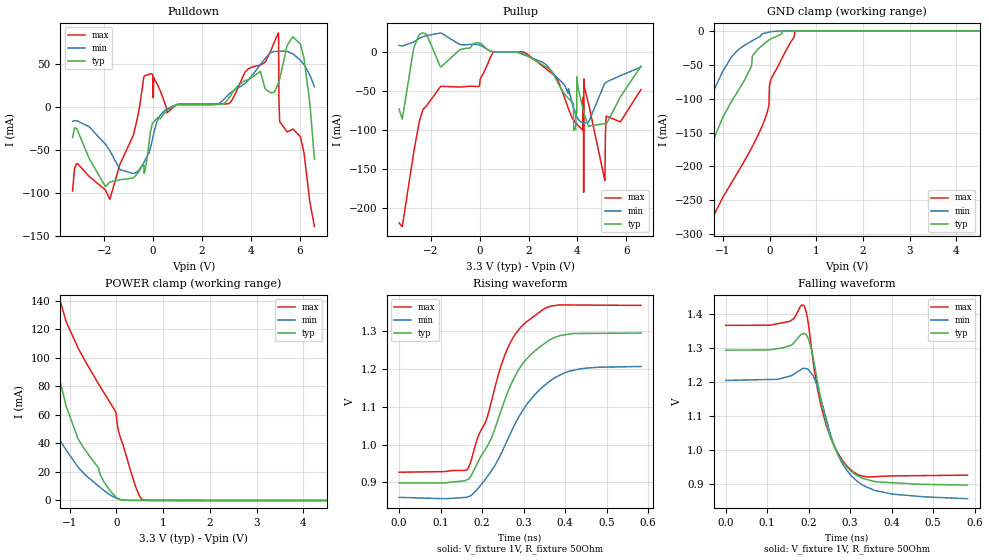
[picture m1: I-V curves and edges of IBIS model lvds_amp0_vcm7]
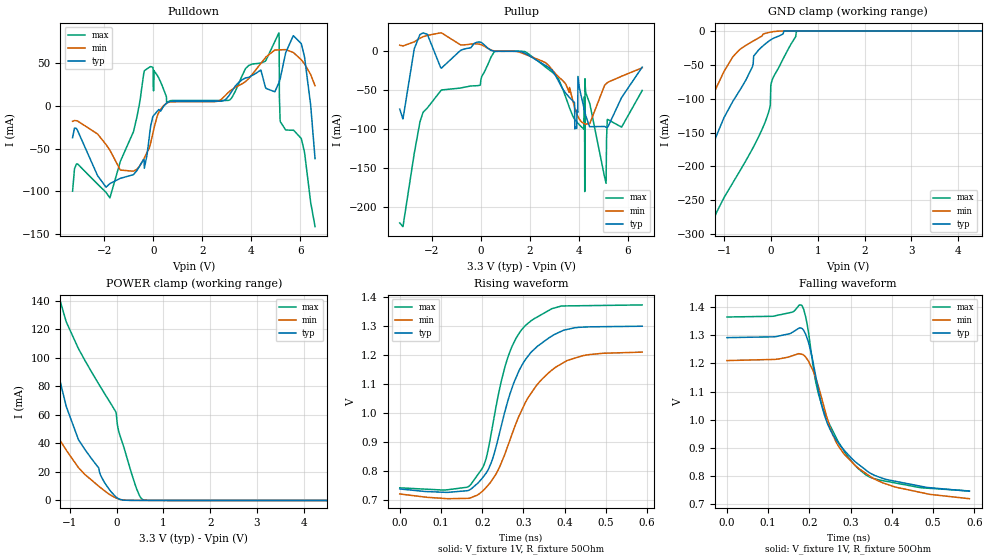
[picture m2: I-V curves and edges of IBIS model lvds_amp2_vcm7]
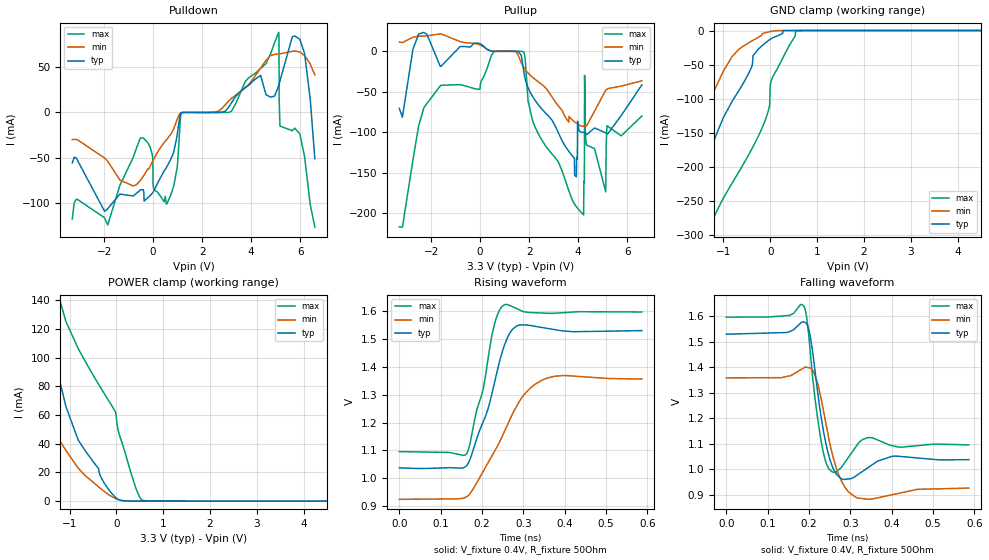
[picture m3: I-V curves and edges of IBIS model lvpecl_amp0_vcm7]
|Texas Instruments Incorporated
| LMK5C33XXX Network Clock Generator/Synchronizer
| Marketing part#   Digital Voltage Range   Package-type   #pins
| LMK5C33216   3.135-3.465V   QFN   64
[IBIS Ver] 4.1
[File name] lmk5c33216.ibs
[File Rev] 1.2
[Date] 2020-10-04
[Source]
| Texas Instruments Incorporated.
| 12500 TI Blvd
| Dallas, TX -75243
[Notes] Revision History:
| Rev 1.2: 2020-10-04, MSG
| - Added models GPIO, XO, INX, I2C for Input/Output pins
| Rev 1.1: 2020-09-02, TT
| - Updated pin names to match datasheet.
| - Corrected typo for LVPECL amplitude names.
| - Note: When AC coupling LVPECL, use small capacitors for best simulation results.
| - Note: When using HSDS, (HSDS_AMP0_VCM7_B0, HSDS_AMP3_VCM7_B0, HSDS_AMP3_VCM7_B1.
| 	- A large deviation in starting voltage may be observed due.
| 	- Setting the common mode voltage may resolve this simulation issue.
| Rev 1.0: 2020-08-25
| - Initial version of the model
| - Model generated from simulations in TISPICE/SPECTRE
| - C_comp although listed in numerical order of value are
| obtained from varying PVT conditions. For PVT conditions for
| each specific value refer the buffer description under
| respective [Model]. IBIS model user is responsible for using
| appropriate C_comp to simulate for Signal Integrity.
| - Warnings regarding combined Non-monotonicity of various models have been
| reviewed and considered minor and can be ignored.
|**** Explanation of [Model Selector]*****************
| - Model names contain the protocol name and
| - amplitude setting 0 to 3 for higher swing
| - DC Shift setting is set to 7
| - HSDS Mode Boost can be on or off as per user requirements
| - lvds_amp0_vcm7 means LVDS MODE, AMPLITUDE 0, DC SHIFT 7
| - hsds_amp0_vcm7_b0 means HSDS MODE, AMPLITUDE 0, DC SHIFT 7, BOOST OFF
| - hsds_amp0_vcm7_b1 means HSDS MODE, AMPLITUDE 0, DC SHIFT 7, BOOST ON
| - cml_amp0_vcm7 means CML MODE, AMPLITUDE 0, DC SHIFT 7
[Disclaimer]
| This model is designed as an aid for customers of Texas Instruments.
| TI and its licensors and suppliers make no warranties, either expressed
| or implied, with respect to this model, including the warranties of
| merchantability or fitness for a particular purpose. The model is
| provided solely on an "as is" basis. The entire risk as to its quality
| and performance is with the customer.
| This model is subject to change without notice. Texas Instruments
| Incorporated is not responsible for updating this model.
[Copyright]
(C) Copyright 2020 Texas Instruments Incorporated. All rights reserved.
| LMK5C33216 (per package)
[Component] LMK5C33216
[Manufacturer] Texas Instruments Incorporated
[Package] |VQFN 64-pin
|   typ   min   max
R_pkg   0.067   0.027   0.083
L_pkg   0.937nH   0.593nH   1.143nH
C_pkg   0.144pF   0.126pF   0.200pF
[Pin]  signal_name 		model_name   R_pin   L_pin   C_pin
1	VDDO_01		power		NA	NA	NA
2	OUT0_P		multimode_out	NA	NA	NA
3	OUT0_N		multimode_out	NA	NA	NA
4	OUT1_P		multimode_out	NA	NA	NA
5	OUT1_N		multimode_out	NA	NA	NA
6	LF1		nc		NA	NA	NA
7	CAP_APLL1		nc		NA	NA	NA
8	VDD_APLL1_XO		power		NA	NA	NA
9	XO_P		xo		NA	NA	NA
10	GPIO2		GPIO		NA	NA	NA
11	VDDO_23		power		NA	NA	NA
12	OUT2_P		multimode_out	NA	NA	NA
13	OUT2_N		multimode_out	NA	NA	NA
14	OUT3_N		multimode_out	NA	NA	NA
15	OUT3_P		multimode_out	NA	NA	NA
16	SDIO		I2C		NA	NA	NA
17	SCK		I2C		NA	NA	NA
18	SCS_ADD_TOD		I2C		NA	NA	NA
19	LF2		nc		NA	NA	NA
20	CAP3_APLL2	nc		NA	NA	NA
21	CAP2_APLL2	nc		NA	NA	NA
22	CAP1_APLL2		nc		NA	NA	NA
23	VDD_APLL2		power		NA	NA	NA
24	OUT5_P		multimode_out	NA	NA	NA
25	OUT5_N		multimode_out	NA	NA	NA
26	OUT4_N		multimode_out	NA	NA	NA
27	OUT4_P		multimode_out	NA	NA	NA
28	VDDO_4567		power		NA	NA	NA
29	OUT6_P		multimode_out	NA	NA	NA
30	OUT6_N		multimode_out	NA	NA	NA
31	OUT7_N		multimode_out	NA	NA	NA
32	OUT7_P		multimode_out	NA	NA	NA
33	VDD_IN0		power		NA	NA	NA
34	IN0_P		INX		NA	NA	NA
35	IN0_N		INX		NA	NA	NA
36	PDN#		I2C		NA	NA	NA
37	VDD_IN1		power		NA	NA	NA
38	IN1_N		INX		NA	NA	NA
39	IN1_P		INX		NA	NA	NA
40	CAP_DIG		nc		NA	NA	NA
41	VDD_DIG		power		NA	NA	NA
42	OUT14_P		multimode_out	NA	NA	NA
43	OUT14_N		multimode_out	NA	NA	NA
44	VDDO_OUT1415		power		NA	NA	NA
45	OUT15_N		multimode_out	NA	NA	NA
46	OUT15_P		multimode_out	NA	NA	NA
47	VDD_APLL3		power		NA	NA	NA
48	CAP_APLL3		nc		NA	NA	NA
49	LF3		nc		NA	NA	NA
50	GPIO0		GPIO		NA	NA	NA
51	OUT8_P		multimode_out	NA	NA	NA
52	OUT8_N		multimode_out	NA	NA	NA
53	OUT9_N		multimode_out	NA	NA	NA
54	OUT9_P		multimode_out	NA	NA	NA
55	VDDO_8910111213	power		NA	NA	NA
56	OUT10_P		multimode_out	NA	NA	NA
57	OUT10_N		multimode_out	NA	NA	NA
58	OUT11_N		multimode_out	NA	NA	NA
59	OUT11_P		multimode_out	NA	NA	NA
60	OUT12_P		multimode_out	NA	NA	NA
61	OUT12_N		multimode_out	NA	NA	NA
62	OUT13_N		multimode_out	NA	NA	NA
63	OUT13_P		multimode_out	NA	NA	NA
64	GPIO1		GPIO		NA	NA	NA
[Diff pin]  inv_pin  vdiff  tdelay_typ  tdelay_min  tdelay_max
2   3   0.0   0.0s   0.0s   0.0s
4   5   0.0   0.0s   0.0s   0.0s
12   13   0.0   0.0s   0.0s   0.0s
14   15   0.0   0.0s   0.0s   0.0s
24   25   0.0   0.0s   0.0s   0.0s
26   27   0.0   0.0s   0.0s   0.0s
29   30   0.0   0.0s   0.0s   0.0s
31   32   0.0   0.0s   0.0s   0.0s
34   35   0.2   0.0s   0.0s   0.0s
38   39   0.2   0.0s   0.0s   0.0s
42   43   0.0   0.0s   0.0s   0.0s
45   46   0.0   0.0s   0.0s   0.0s
51   52   0.0   0.0s   0.0s   0.0s
53   54   0.0   0.0s   0.0s   0.0s
56   57   0.0   0.0s   0.0s   0.0s
58   59   0.0   0.0s   0.0s   0.0s
60   61   0.0   0.0s   0.0s   0.0s
62   63   0.0   0.0s   0.0s   0.0s
|CML MODE available only on pins Out4 & 6 and not available on any other pins
[Model Selector] multimode_out
lvds_amp0_vcm7 Amplitude setting 0, DC shift setting 7
lvds_amp1_vcm7 Amplitude setting 1, DC shift setting 7
lvds_amp2_vcm7 Amplitude setting 2, DC shift setting 7
lvds_amp3_vcm7 Amplitude setting 3, DC shift setting 7
lvpecl_amp0_vcm7 Amplitude setting 0, DC shift setting 7
lvpecl_amp1_vcm7 Amplitude setting 1, DC shift setting 7
lvpecl_amp2_vcm7 Amplitude setting 2, DC shift setting 7
lvpecl_amp3_vcm7 Amplitude setting 3, DC shift setting 7
hsds_amp0_vcm7_b0 Amplitude setting 0, DC shift setting 7, Boost off
hsds_amp0_vcm7_b1 Amplitude setting 0, DC shift setting 7, Boost on
hsds_amp1_vcm7_b0 Amplitude setting 1, DC shift setting 7, Boost off
hsds_amp1_vcm7_b1 Amplitude setting 1, DC shift setting 7, Boost on
hsds_amp2_vcm7_b0 Amplitude setting 2, DC shift setting 7, Boost off
hsds_amp2_vcm7_b1 Amplitude setting 2, DC shift setting 7, Boost on
hsds_amp3_vcm7_b0 Amplitude setting 3, DC shift setting 7, Boost off
hsds_amp3_vcm7_b1 Amplitude setting 3, DC shift setting 7, Boost on
cml_amp0_vcm7 Amplitude setting 0, DC shift setting 7
cml_amp1_vcm7 Amplitude setting 1, DC shift setting 7
cml_amp2_vcm7 Amplitude setting 2, DC shift setting 7
cml_amp3_vcm7 Amplitude setting 3, DC shift setting 7
[Model Selector] GPIO
GPIO_IO   3.3V   digital I/O
GPIO_OD   3.3V   digital Open_drain
| Models and submodels in the file (25): lvds_amp0_vcm7 (Output), lvds_amp1_vcm7 (Output), lvds_amp2_vcm7 (Output), lvds_amp3_vcm7 (Output), lvpecl_amp0_vcm7 (Output), lvpecl_amp1_vcm7 (Output), lvpecl_amp2_vcm7 (Output), lvpecl_amp3_vcm7 (Output), hsds_amp0_vcm7_b0 (Output), hsds_amp0_vcm7_b1 (Output), hsds_amp1_vcm7_b0 (Output), hsds_amp1_vcm7_b1 (Output), hsds_amp2_vcm7_b0 (Output), hsds_amp2_vcm7_b1 (Output), hsds_amp3_vcm7_b0 (Output), hsds_amp3_vcm7_b1 (Output), cml_amp0_vcm7 (Output), cml_amp1_vcm7 (Output), cml_amp2_vcm7 (Output), cml_amp3_vcm7 (Output), GPIO_IO (I/O), GPIO_OD (I/O_open_drain), I2C (I/O_open_drain), xo (Input), INX (Input)
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[Model]   lvds_amp0_vcm7
Model_type   Output
Polarity   Non-Inverting
Vmeas = 1.1
Vref = 1
Cref = 0pF
Rref = 50
|   typ   min   max
C_comp   0.65pF   0.575pF   0.725pF
[Voltage Range]   3.3   3.135   3.465
[Temperature Range]   50   135   -40
[Pullup Reference]   3.3   3.135   3.465
[Pulldown Reference]   0   0   0
[Power Clamp Reference]   3.3   3.135   3.465
[GND Clamp Reference]   0   0   0
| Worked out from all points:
|   slope of the pulldown table from 0 to 0.495 V, typ, clamps not added: 42.2 ohm
|   slope of the pullup table from 0 to 0.495 V, typ, clamps not added: 45.5 ohm
|   falling waveform, V_fixture 1V, R_fixture 50Ohm: 20-80 % time 56.5ps typ, 68.5ps min, 52ps max; typ from 1.29 V to 0.898 V
|   rising waveform, V_fixture 1V, R_fixture 50Ohm: 20-80 % time 97ps typ, 110ps min, 84.5ps max; typ from 0.898 V to 1.29 V
[Pulldown]
|   Voltage   I(typ)   I(min)   I(max)
-3.3V     -35.3mA    -16.44mA   -97.86mA
-3.092V   -27.25mA   -16.11mA   -65.86mA
-1.775V   -87.34mA   -50.64mA   -107.5mA
-815.1mV  -82.57mA   -77.39mA   -32.84mA
-349.8mV  -75.39mA   -62.8mA    36.81mA
214.5mV   -11.39mA   -12.84mA   24.09mA
3.066V    9.309mA    14.38mA    4.089mA
5.125V    28.22mA    65.42mA    86.96mA
5.145V    30.01mA    65.45mA    12.02mA
5.184V    34.01mA    65.52mA    -16.96mA
6.026V    73.78mA    54.84mA    -34.39mA
6.6V      -60.59mA   23.95mA    -139.3mA
[GND Clamp]
|   Voltage   I(typ)   I(min)   I(max)
-3.3V     -892.9mA   -765.6mA   -1.068A
-1.924V   -314.6mA   -288.5mA   -459.9mA
-1.815V   -287mA     -251.4mA   -425.6mA
-1.478V   -218.2mA   -143.5mA   -333.1mA
-1.162V   -154.3mA   -82.94mA   -268mA
-815.1mV  -104mA     -38.12mA   -224.4mA
-171.6mV  -22.09mA   -4.573mA   -142.5mA
-13.2mV   -13.46mA   -1.685mA   -109.6mA
-3.3mV    -13.01mA   -1.546mA   -81.32mA
26.4mV    -11.77mA   -1.169mA   -72.31mA
551.1mV   0A         -83.65nA   -742.8uA
6.6V      0A         0A         0A
[Pullup]
|   Voltage   I(typ)   I(min)   I(max)
-3.3V     -73.12mA   8.337mA    -218.6mA
-2.32V    24.27mA    19.34mA    -73.75mA
561mV     41.56uA    225uA      -562.9uA
3.066V    -31.59mA   -29.52mA   -30.42mA
4.224V    -72.71mA   -90.79mA   -100mA
4.234V    -74.02mA   -90.87mA   -58.22mA
4.244V    -75.33mA   -90.93mA   -59.25mA
4.254V    -76.63mA   -90.99mA   -179.5mA
4.264V    -77.93mA   -91.04mA   -34.69mA
5.125V    -91.98mA   -40.34mA   -164.3mA
5.174V    -91.84mA   -38.96mA   -82.61mA
6.6V      -18.44mA   -19.42mA   -48.2mA
[POWER Clamp]
|   Voltage   I(typ)   I(min)   I(max)
-3.3V     330.7mA    180mA      566.4mA
-2.736V   200mA      135.8mA    401.6mA
-1.647V   138.3mA    65.17mA    197.7mA
-1.459V   117.6mA    55.06mA    168.7mA
-1.082V   66.76mA    35.64mA    126mA
-815.1mV  42.67mA    23.06mA    106.5mA
-3.3mV    2.23mA     1.644mA    59.85mA
46.2mV    1.16mA     1.045mA    48.47mA
313.5mV   86.42uA    94.45uA    19.62mA
491.7mV   74.41uA    72.76uA    3.272mA
570.9mV   69.96uA    68.47uA    464.6uA
6.6V      0A         0A         0A
[Ramp]
R_load = 50
|   typ   min   max
dV/dt_r   0.2377/9.71594e-11   0.207333/1.09667e-10   0.264262/8.45933e-11
dV/dt_f   0.237632/5.65009e-11   0.208363/6.82135e-11   0.263927/5.1862e-11
[Falling Waveform]
V_fixture = 1V
V_fixture_min = 0.95V
V_fixture_max = 1.05V
R_fixture = 50Ohm
C_fixture = 0F
|   Time   V(typ)   V(min)   V(max)
0s        1.294V     1.205V     1.367V
153ps     1.307V     1.217V     1.379V
187.1ps   1.342V     1.241V     1.426V
204.7ps   1.307V     1.229V     1.321V
218.9ps   1.218V     1.195V     1.197V
236.2ps   1.111V     1.121V     1.101V
260.9ps   1.013V     1.017V     1.016V
292.5ps   951.4mV    940.8mV    953.9mV
358.3ps   908.7mV    882.8mV    922.7mV
582.7ps   898.3mV    858.2mV    927.3mV
[Rising Waveform]
V_fixture = 1V
V_fixture_min = 0.95V
V_fixture_max = 1.05V
R_fixture = 50Ohm
C_fixture = 0F
|   Time   V(typ)   V(min)   V(max)
0s        898.4mV    860.7mV    927.1mV
164.8ps   907.6mV    861.8mV    935.4mV
220.9ps   1.013V     928.2mV    1.107V
242.5ps   1.079V     968.8mV    1.197V
264.6ps   1.146V     1.02V      1.262V
300.5ps   1.218V     1.095V     1.318V
345.2ps   1.263V     1.151V     1.356V
387.8ps   1.288V     1.184V     1.369V
435.7ps   1.293V     1.2V       1.369V
582.7ps   1.295V     1.206V     1.368V
[Model]   lvds_amp2_vcm7
Model_type   Output
Polarity   Non-Inverting
Vmeas = 1
Vref = 1
Cref = 0pF
Rref = 50
|   typ   min   max
C_comp   0.65pF   0.575pF   0.725pF
[Voltage Range]   3.3   3.135   3.465
[Temperature Range]   50   135   -40
[Pullup Reference]   3.3   3.135   3.465
[Pulldown Reference]   0   0   -0
[Power Clamp Reference]   3.3   3.135   3.465
[GND Clamp Reference]   0   0   0
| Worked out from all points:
|   slope of the pulldown table from 0 to 0.495 V, typ, clamps not added: 36.4 ohm
|   slope of the pullup table from 0 to 0.495 V, typ, clamps not added: 44.9 ohm
|   falling waveform, V_fixture 1V, R_fixture 50Ohm: 20-80 % time 96.1ps typ, 106ps min, 88.4ps max; typ from 1.29 V to 0.747 V
|   rising waveform, V_fixture 1V, R_fixture 50Ohm: 20-80 % time 79.2ps typ, 98.5ps min, 64.6ps max; typ from 0.738 V to 1.3 V
[Pulldown]
|   Voltage   I(typ)   I(min)   I(max)
-3.3V     -37.26mA   -18.13mA   -99.9mA
-3.102V   -28.57mA   -17.7mA    -67.86mA
-1.775V   -90.99mA   -51.93mA   -107.7mA
-815.1mV  -80.51mA   -76.49mA   -30.4mA
-260.7mV  -57.56mA   -54.29mA   43.27mA
551.1mV   3.222mA    3.219mA    3.835mA
3.066V    11.13mA    15.76mA    6.362mA
5.125V    26.86mA    65.39mA    85.34mA
5.145V    28.63mA    65.42mA    10.32mA
5.184V    32.58mA    65.48mA    -18.74mA
6.036V    72.73mA    53.9mA     -38.22mA
6.6V      -61.84mA   23.44mA    -141.3mA
[GND Clamp]
|   Voltage   I(typ)   I(min)   I(max)
-3.3V     -892.9mA   -765.6mA   -1.068A
-1.924V   -314.6mA   -288.5mA   -459.9mA
-1.815V   -287mA     -251.4mA   -425.6mA
-1.478V   -218.2mA   -143.5mA   -333.1mA
-1.162V   -154.3mA   -82.94mA   -268mA
-815.1mV  -104mA     -38.12mA   -224.4mA
-171.6mV  -22.09mA   -4.573mA   -142.5mA
-13.2mV   -13.46mA   -1.685mA   -109.6mA
-3.3mV    -13.01mA   -1.546mA   -81.32mA
26.4mV    -11.77mA   -1.169mA   -72.31mA
551.1mV   0A         -83.65nA   -742.8uA
6.6V      0A         0A         0A
[Pullup]
|   Voltage   I(typ)   I(min)   I(max)
-3.3V     -73.95mA   7.799mA    -219.8mA
-2.35V    23.53mA    18.61mA    -78.25mA
-1.597V   -21.59mA   23.57mA    -49.56mA
561mV     96.81uA    380.9uA    -554.2uA
4.224V    -73.06mA   -92.53mA   -99.94mA
4.234V    -74.41mA   -92.66mA   -58.14mA
4.244V    -75.76mA   -92.78mA   -59.17mA
4.254V    -77.11mA   -92.89mA   -179.7mA
4.264V    -78.45mA   -92.99mA   -35.12mA
5.125V    -97.28mA   -41.67mA   -169mA
5.174V    -97.28mA   -40.31mA   -87.6mA
6.6V      -20.28mA   -21.13mA   -50.18mA
[POWER Clamp]
|   Voltage   I(typ)   I(min)   I(max)
-3.3V     330.7mA    180mA      566.4mA
-2.736V   200mA      135.8mA    401.6mA
-1.647V   138.3mA    65.17mA    197.7mA
-1.459V   117.6mA    55.06mA    168.7mA
-1.082V   66.76mA    35.64mA    126mA
-815.1mV  42.67mA    23.06mA    106.5mA
-3.3mV    2.23mA     1.644mA    59.85mA
46.2mV    1.16mA     1.045mA    48.47mA
313.5mV   86.42uA    94.45uA    19.62mA
491.7mV   74.41uA    72.76uA    3.272mA
570.9mV   69.96uA    68.47uA    464.6uA
6.6V      0A         0A         0A
[Ramp]
R_load = 50
|   typ   min   max
dV/dt_r   0.336634/7.90854e-11   0.293455/9.84312e-11   0.378383/6.42045e-11
dV/dt_f   0.326314/9.60134e-11   0.293455/1.04642e-10   0.369558/8.79734e-11
[Falling Waveform]
V_fixture = 1V
V_fixture_min = 0.95V
V_fixture_max = 1.05V
R_fixture = 50Ohm
C_fixture = 0F
|   Time   V(typ)   V(min)   V(max)
0s        1.291V     1.21V      1.364V
111.1ps   1.294V     1.213V     1.366V
181ps     1.324V     1.232V     1.406V
199.1ps   1.267V     1.203V     1.296V
215.2ps   1.156V     1.149V     1.135V
230.8ps   1.045V     1.071V     1.048V
265.1ps   928.8mV    920.3mV    936mV
304.8ps   860mV      847.7mV    847.9mV
405.8ps   783mV      762.9mV    776.8mV
588ps     746.9mV    720.5mV    747.9mV
[Rising Waveform]
V_fixture = 1V
V_fixture_min = 0.95V
V_fixture_max = 1.05V
R_fixture = 50Ohm
C_fixture = 0F
|   Time   V(typ)   V(min)   V(max)
0s        737.8mV    720.5mV    741.6mV
172.5ps   737.3mV    707.6mV    753.8mV
208ps     789.7mV    740.6mV    835.6mV
225.3ps   842.3mV    771.6mV    956.9mV
244.9ps   947mV      822.8mV    1.101V
267.1ps   1.064V     905.9mV    1.211V
289.2ps   1.145V     989mV      1.273V
319.1ps   1.21V      1.069V     1.318V
405.8ps   1.288V     1.181V     1.369V
588ps     1.299V     1.21V      1.372V
[Model]   lvpecl_amp0_vcm7
Model_type   Output
Polarity   Non-Inverting
Vmeas = 1.3
Vref = 0.4
Cref = 0pF
Rref = 50
|   typ   min   max
C_comp   0.65pF   0.575pF   0.725pF
[Voltage Range]   3.3   3.135   3.465
[Temperature Range]   50   135   -40
[Pullup Reference]   3.3   3.135   3.465
[Pulldown Reference]   0   0   0
[Power Clamp Reference]   3.3   3.135   3.465
[GND Clamp Reference]   0   0   0
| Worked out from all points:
|   slope of the pulldown table from 0 to 0.495 V, typ, clamps not added: 19.8 ohm
|   slope of the pullup table from 0 to 0.495 V, typ, clamps not added: 52.7 ohm
|   falling waveform, V_fixture 0.4V, R_fixture 50Ohm: 20-80 % time 25.4ps typ, 34.6ps min, 20.3ps max; typ from 1.53 V to 1.04 V
|   rising waveform, V_fixture 0.4V, R_fixture 50Ohm: 20-80 % time 58.6ps typ, 90.5ps min, 41.6ps max; typ from 1.04 V to 1.53 V
[Pulldown]
|   Voltage   I(typ)   I(min)   I(max)
-3.3V     -55.76mA   -29.95mA   -117.6mA
-1.855V   -106.3mA   -53.89mA   -124.2mA
-676.5mV  -89.25mA   -79.63mA   -39.08mA
541.2mV   -60.71mA   -30.31mA   -101.3mA
976.8mV   -25.99mA   -7.952mA   -61.37mA
1.155V    -389.8uA   -236.2uA   -663.5uA
3.165V    9.137mA    14.64mA    773.6uA
5.125V    29.54mA    64.47mA    88.37mA
5.145V    31.43mA    64.54mA    13.51mA
5.184V    35.59mA    64.67mA    -15.14mA
5.986V    80.77mA    66.7mA     -23.68mA
6.6V      -51.17mA   41.43mA    -126.6mA
[GND Clamp]
|   Voltage   I(typ)   I(min)   I(max)
-3.3V     -892.9mA   -765.6mA   -1.068A
-1.924V   -314.6mA   -288.5mA   -459.9mA
-1.815V   -287mA     -251.4mA   -425.6mA
-1.478V   -218.2mA   -143.5mA   -333.1mA
-1.162V   -154.3mA   -82.94mA   -268mA
-815.1mV  -104mA     -38.12mA   -224.4mA
-171.6mV  -22.09mA   -4.573mA   -142.5mA
-13.2mV   -13.46mA   -1.685mA   -109.6mA
-3.3mV    -13.01mA   -1.546mA   -81.32mA
26.4mV    -11.77mA   -1.169mA   -72.35mA
551.1mV   0A         -83.65nA   -744.1uA
6.6V      0A         0A         0A
[Pullup]
|   Voltage   I(typ)   I(min)   I(max)
-3.3V     -70.4mA    11.48mA    -216.8mA
-2.3V     23.4mA     18.77mA    -70.17mA
570.9mV   -35.9uA    22.68uA    -439.4uA
1.789V    -26.35mA   -20.62mA   -1.29mA
3.858V    -153.3mA   -87.27mA   -189mA
4.224V    -100.2mA   -92.64mA   -202.1mA
4.254V    -100.4mA   -92.57mA   -162.3mA
4.264V    -100.6mA   -92.54mA   -29.75mA
4.333V    -102.7mA   -92.26mA   -114.8mA
5.125V    -100.8mA   -48.21mA   -173.6mA
5.174V    -102.1mA   -46.98mA   -92.64mA
6.6V      -41.59mA   -36.46mA   -79.98mA
[POWER Clamp]
|   Voltage   I(typ)   I(min)   I(max)
-3.3V     330.7mA    180mA      566.4mA
-2.736V   200mA      135.8mA    401.6mA
-1.647V   138.3mA    65.17mA    197.7mA
-1.459V   117.6mA    55.06mA    168.7mA
-1.082V   66.76mA    35.64mA    126mA
-815.1mV  42.67mA    23.06mA    106.5mA
-3.3mV    2.23mA     1.644mA    59.85mA
46.2mV    1.16mA     1.045mA    48.48mA
313.5mV   86.42uA    94.45uA    19.62mA
491.7mV   74.41uA    72.76uA    3.271mA
570.9mV   69.96uA    68.47uA    464.4uA
6.6V      0A         0A         0A
[Ramp]
R_load = 50
|   typ   min   max
dV/dt_r   0.294996/5.87219e-11   0.258764/9.06663e-11   0.300287/4.16354e-11
dV/dt_f   0.294996/2.53774e-11   0.259206/3.44885e-11   0.300287/2.01414e-11
[Falling Waveform]
V_fixture = 0.4V
V_fixture_min = 0.35V
V_fixture_max = 0.45V
R_fixture = 50Ohm
C_fixture = 0F
|   Time   V(typ)   V(min)   V(max)
0s        1.53V      1.359V     1.596V
187.3ps   1.578V     1.397V     1.64V
195ps     1.568V     1.399V     1.589V
203ps     1.523V     1.397V     1.463V
227.8ps   1.222V     1.289V     1.126V
256.1ps   1.013V     1.062V     990mV
286.3ps   960.8mV    931.3mV    1.026V
317.6ps   978.8mV    887.5mV    1.098V
401.2ps   1.051V     900.5mV    1.093V
586.5ps   1.038V     926.5mV    1.096V
[Rising Waveform]
V_fixture = 0.4V
V_fixture_min = 0.35V
V_fixture_max = 0.45V
R_fixture = 50Ohm
C_fixture = 0F
|   Time   V(typ)   V(min)   V(max)
0s        1.038V     924.8mV    1.096V
163.4ps   1.047V     934.8mV    1.09V
203.1ps   1.204V     1.026V     1.322V
230.5ps   1.344V     1.098V     1.554V
253.5ps   1.474V     1.166V     1.622V
271ps     1.529V     1.222V     1.617V
286.9ps   1.548V     1.267V     1.606V
317.6ps   1.548V     1.324V     1.594V
353.4ps   1.539V     1.357V     1.592V
586.5ps   1.53V      1.356V     1.596V
